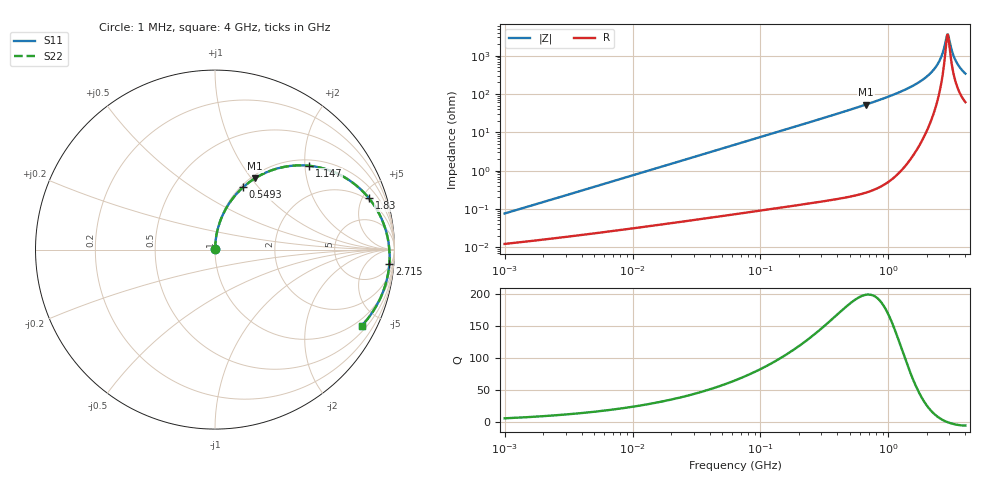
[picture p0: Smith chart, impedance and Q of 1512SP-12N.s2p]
# MHz  S  MA  R  50
!Freq  MagS11  AngS11  MagS21  AngS21  MagS12  AngS12  MagS22  AngS22
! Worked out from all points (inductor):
!   801 points, 1 MHz to 4 GHz, reference 50 ohm
!   read as one part in series: L = 11.9 nH near 1.042 MHz
!   highest Q = 199 at 669 MHz (marker M1), where L = 12.6 nH
!   self-resonance near 2.889 GHz
!   S11 on the Smith chart (normalised r, x): 1 MHz: 1.00, +0.00; 549.3 MHz: 1.03, +0.84; 1.147 GHz: 1.14, +2.10; 1.83 GHz: 1.78, +5.60; 2.715 GHz: 7, -23; 4 GHz: 0.71, -3.98
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1  0.0007353 80.4  0.9999 -0.0  0.9999 -0.0  0.0007353 80.4
4.016383  0.002919 85.7  0.9998 -0.2  0.9998 -0.2  0.002919 85.7
15.96482  0.01158 87.4  0.9996 -0.7  0.9996 -0.7  0.01158 87.4
63.45894  0.04597 86.3  0.9982 -2.8  0.9982 -2.8  0.04596 86.3
252.2445  0.1811 78.4  0.9821 -11.1  0.9821 -11.1  0.1811 78.4
549.2741  0.3817 65.7  0.9223 -24.0  0.9223 -24.0  0.3816 65.7
668.9713  0.4559 60.7  0.8877 -29.0  0.8877 -29.0  0.4558 60.7
1013.11  0.6419 46.8  0.7629 -42.8  0.7629 -42.8  0.6417 46.8
1147.444  0.7022 41.7  0.7069 -47.9  0.7069 -47.9  0.702 41.7
1456.716  0.8144 30.6  0.5703 -58.7  0.5703 -58.7  0.8141 30.6
1830.257  0.9043 18.5  0.4035 -70.0  0.4035 -70.0  0.904 18.5
2094.561  0.9426 10.8  0.2914 -76.4  0.2914 -76.4  0.9424 10.8
2347.803  0.9638 4.1  0.1917 -80.6  0.1917 -80.6  0.9637 4.1
2551.006  0.9722 -0.8  0.1185 -80.7  0.1185 -80.7  0.9722 -0.8
2714.869  0.9745 -4.6  0.0654 -73.4  0.0654 -73.4  0.9745 -4.6
2829.918  0.9742 -7.1  0.03512 -50.6  0.03512 -50.6  0.9742 -7.1
2889.257  0.9734 -8.3  0.02711 -20.9  0.02711 -20.9  0.9735 -8.3
2949.842  0.9723 -9.5  0.03008 14.5  0.03008 14.5  0.9725 -9.5
3205.151  0.9645 -14.5  0.0893 54.6  0.0893 54.6  0.9648 -14.5
3375.823  0.957 -17.6  0.1311 57.1  0.1311 57.1  0.9574 -17.6
3668.002  0.9413 -22.4  0.1962 55.9  0.1962 55.9  0.9419 -22.4
4000  0.9208 -27.4  0.2598 52.5  0.2598 52.5  0.9217 -27.4
